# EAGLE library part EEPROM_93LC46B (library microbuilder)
1K 16-Bit EEPROM (Compatible with FT2232H) SOIC8 - Digikey: 93LC46BT-I/SNCT-ND
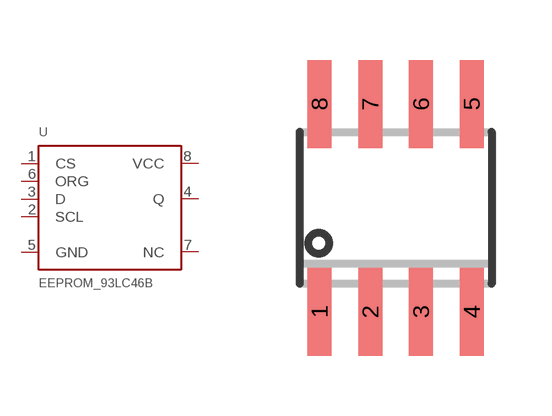
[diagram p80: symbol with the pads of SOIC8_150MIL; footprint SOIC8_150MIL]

Designator prefix U

## EEPROM_93LC46B  [SOIC8_150MIL]
1  CS  in
2  SCL  in
3  D  in
4  Q  out
5  GND  pwr
6  ORG
7  NC  nc
8  VCC  pwr

## Footprint SOIC8_150MIL (pad centres in mm)
Small Outline IC - 150mil Wide
smd 0.6 x 2.2: 1 -1.905,-2.6; 2 -0.635,-2.6; 3 0.635,-2.6; 4 1.905,-2.6; 5 1.905,2.6; 6 0.635,2.6; 7 -0.635,2.6; 8 -1.905,2.6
